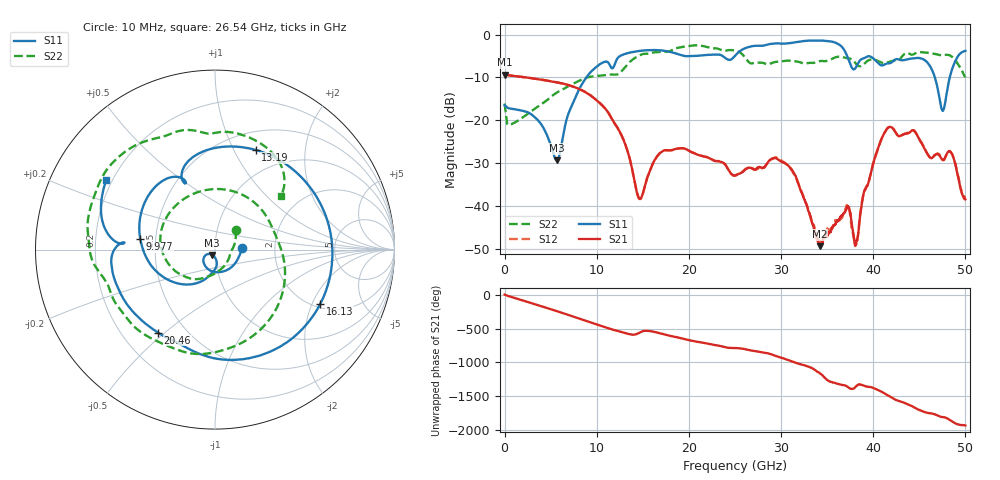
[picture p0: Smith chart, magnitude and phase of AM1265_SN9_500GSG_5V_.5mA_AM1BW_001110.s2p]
!Keysight Technologies,N5245B,MY58422270,A.16.20.02
!Date: Thursday, March 05, 2026 00:45:59
!Correction: S11(C  2-Port  )
!S21(C  2-Port  )
!S12(C  2-Port  )
!S22(C  2-Port  )
!S2P File: Measurements: S11, S21, S12, S22:
# Hz S  dB  R 50
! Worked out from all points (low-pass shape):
!   3201 points, 10 MHz to 50 GHz, reference 50 ohm
!   highest |S21| = -9.36 dB at 10 MHz (marker M1); lowest = -49.4 dB at 34.22 GHz (marker M2)
!   |S21| within 3 dB of the highest: start of sweep to 7.714 GHz
!   lowest |S11| = -29.4 dB at 5.681 GHz (marker M3), VSWR 1.07, Z = 48.3 - j2.87 ohm
!   |S11| at or under -10 dB: start of sweep to 8.883 GHz; 46.69 GHz to 48.3 GHz (1.614 GHz wide, 3.4 % of centre)
!   |S22| runs from -21.1 to -2.5 dB; largest |S21 - S12| = 0.0056
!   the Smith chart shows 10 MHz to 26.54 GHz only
!   S11 on the Smith chart (normalised r, x): 10 MHz: 1.35, +0.02; 9.977 GHz: 0.41, +0.06; 13.19 GHz: 0.71, +1.22; 16.13 GHz: 2.17, -2.31; 20.46 GHz: 0.35, -0.47; 26.54 GHz: 0.18, +0.28
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1e7  -16.48 2.7  -9.36 4.0  -9.48 3.5  -16.10 43.1
2.306416e9  -17.97 -86.6  -9.99 -97.7  -9.99 -97.7  -18.85 -73.1
5.680741e9  -29.39 -118.8  -11.16 118.0  -11.16 118.0  -13.54 -130.0
8.352081e9  -11.77 -131.1  -12.96 -3.3  -12.94 -3.3  -10.53 179.7
9.976756e9  -7.53 172.0  -15.32 -77.6  -15.31 -77.7  -9.66 130.9
1.319486e10  -4.44 67.9  -26.21 148.4  -26.16 148.3  -7.31 -26.4
1.46477e10  -3.82 18.8  -38.39 159.0  -38.33 158.4  -4.87 -89.4
1.613178e10  -3.61 -27.1  -29.93 174.5  -29.98 174.5  -4.17 -132.6
1.667854e10  -3.64 -43.0  -28.09 156.4  -28.09 156.3  -4.12 -145.0
2.045903e10  -5.02 -124.6  -27.59 36.0  -27.62 36.3  -2.56 149.6
2.5005e10  -4.97 174.9  -32.93 -68.4  -32.86 -68.4  -3.75 70.4
2.653594e10  -2.88 147.5  -31.07 -98.9  -31.14 -98.9  -6.50 39.4
3.066012e10  -2.09 79.0  -30.38 118.9  -30.36 119.8  -6.09 -55.3
3.334708e10  -1.40 35.7  -43.91 -5.2  -43.55 -4.7  -6.62 -133.3
3.422191e10  -1.38 20.4  -49.39 -83.0  -48.53 -91.6  -6.18 -152.4
3.717444e10  -5.01 -40.9  -40.24 81.4  -39.98 77.5  -5.51 149.9
3.815862e10  -7.52 -23.1  -48.27 87.8  -48.68 87.4  -6.89 133.8
4.167354e10  -6.72 -54.0  -21.66 -57.4  -21.61 -57.9  -6.41 110.2
4.515722e10  -5.54 -101.9  -25.07 84.2  -24.92 83.8  -4.09 73.4
4.656319e10  -9.21 -151.1  -28.39 34.6  -28.36 34.2  -4.47 54.1
4.770358e10  -17.02 68.7  -29.12 -14.7  -29.20 -15.4  -4.77 41.7
5e10  -3.80 -72.0  -38.45 -135.7  -37.66 -121.0  -9.98 8.7
